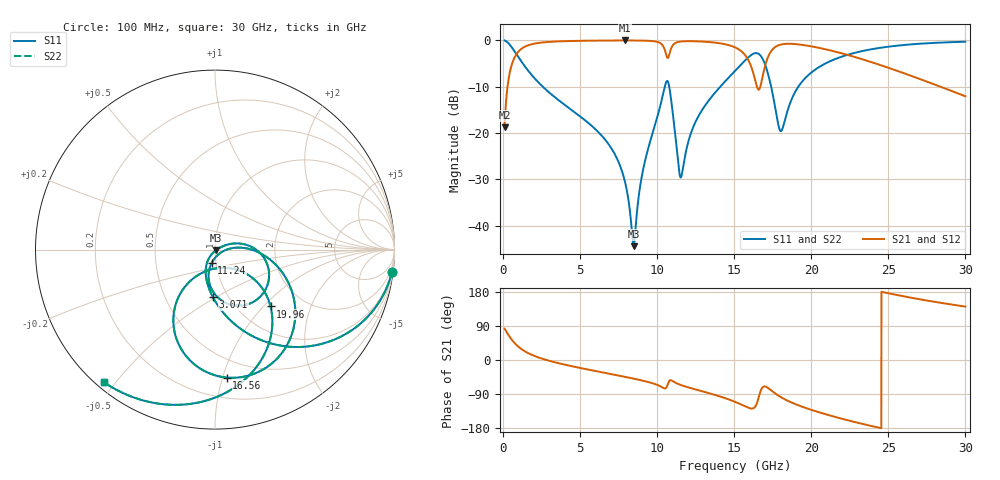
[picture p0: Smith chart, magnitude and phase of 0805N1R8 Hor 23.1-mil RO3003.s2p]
# GHz S MA R 50
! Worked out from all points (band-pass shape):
!   3201 points, 100 MHz to 30 GHz, reference 50 ohm
!   highest |S21| = -0.05 dB at 7.911 GHz (marker M1); lowest = -18.8 dB at 100 MHz (marker M2)
!   |S21| within 3 dB of the highest: 861 MHz to 10.58 GHz (9.72 GHz wide, 170 % of centre); 17.27 GHz to 22.22 GHz (4.952 GHz wide, 25.1 % of centre)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
!   lowest |S11| = -44.5 dB at 8.472 GHz (marker M3), VSWR 1.01, Z = 50.4 - j0.474 ohm
!   |S11| at or under -10 dB: 2.567 GHz to 10.5 GHz (7.929 GHz wide, 121 % of centre); 10.78 GHz to 14.1 GHz (3.321 GHz wide, 26.7 % of centre); 17.39 GHz to 19.16 GHz (1.772 GHz wide, 9.7 % of centre)
!   |S22| runs from -44.5 to -0.1 dB; largest |S21 - S12| = 0
!   S11 on the Smith chart (normalised r, x): 100 MHz: 1, -16; 3.071 GHz: 0.85, -0.49; 11.24 GHz: 0.95, -0.14; 16.56 GHz: 0.35, -1.03; 19.96 GHz: 1.39, -1.10; 30 GHz: 0.02, -0.47
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0.1  0.9934 -7.2  0.1144 82.8  0.1144 82.8  0.9934 -7.2
0.4176875  0.901 -28.2  0.4335 61.8  0.4335 61.8  0.901 -28.2
0.8381563  0.7188 -49.0  0.6943 40.9  0.6943 40.9  0.7188 -49.0
3.071312  0.2659 -92.5  0.9618 -2.9  0.9618 -2.9  0.2659 -92.5
5.089563  0.1467 -110.6  0.986 -21.7  0.986 -21.7  0.1467 -110.6
7.911375  0.02961 -124.8  0.9943 -44.4  0.9943 -44.4  0.02961 -124.8
8.472  0.005988 -51.7  0.9937 -49.1  0.9937 -49.1  0.005988 -51.7
9.07  0.0389 23.2  0.9907 -54.6  0.9907 -54.6  0.0389 23.2
10.06978  0.1616 10.9  0.9529 -66.8  0.9529 -66.8  0.1616 10.9
10.68647  0.3597 -55.6  0.6424 -64.0  0.6424 -64.0  0.3597 -55.6
11.23775  0.07551 -103.8  0.943 -60.9  0.943 -60.9  0.07551 -103.8
11.56478  0.0338 -39.4  0.9694 -66.4  0.9694 -66.4  0.0338 -39.4
12.62063  0.1453 4.3  0.9726 -79.2  0.9726 -79.2  0.1453 4.3
15.05  0.4666 -26.2  0.8376 -110.4  0.8376 -110.4  0.4666 -26.2
15.93766  0.6581 -51.4  0.6003 -126.3  0.6003 -126.3  0.6581 -51.4
16.56369  0.7158 -84.8  0.293 -102.0  0.293 -102.0  0.7158 -84.8
17.13366  0.4683 -119.7  0.6218 -72.1  0.6218 -72.1  0.4683 -119.7
18.02131  0.1045 -82.9  0.8981 -97.9  0.8981 -97.9  0.1045 -82.9
19.96481  0.4429 -45.7  0.8609 -131.0  0.8609 -131.0  0.4429 -45.7
20.03956  0.4532 -46.5  0.8564 -132.0  0.8564 -132.0  0.4532 -46.5
25.01978  0.8525 -95.3  0.5031 176.0  0.5031 176.0  0.8525 -95.3
30  0.9639 -129.9  0.2483 141.0  0.2483 141.0  0.9639 -129.9
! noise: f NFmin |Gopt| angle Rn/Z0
0.1  0.001089  0.9458  1.424  0.004504
3.417  0.006774  0.7223  21.14  0.004678
6.743  0.0121  0.7041  39.87  0.007116
10.06  0.04295  0.8687  57.59  0.05411
13.39  0.03543  0.8038  74.33  0.02398
16.7  0.4097  0.9777  90.4  2.077
20.03  0.06208  0.8412  104.7  0.03133
23.35  0.06063  0.8198  117.4  0.01951
26.67  0.07285  0.8351  129.7  0.01748
30  0.09506  0.8639  141.7  0.01685
